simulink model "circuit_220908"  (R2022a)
settings: Solver=VariableStepAuto  StartTime=-D+0.1e-6  StopTime=34e-6  FixedStep=1e-3  MaxStep=0.1e-6  RelTol=1e-3
model workspace (MATLAB code in the model file):
  sGeo = CreateGeometry()
  sConst = CreateConstants()
libraries: fl_lib x14, nesl_utility x3, ee_lib x1

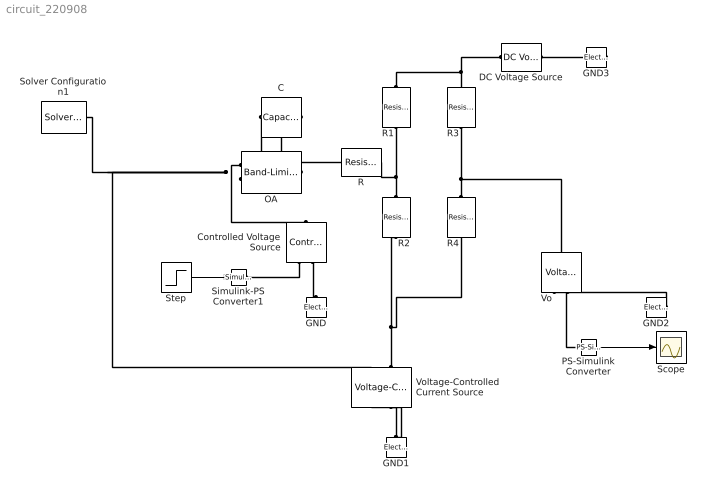
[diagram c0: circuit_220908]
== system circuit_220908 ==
  C : fl_lib/Electrical/Electrical Elements/Capacitor  c=20 nF  r=0 Ohm  g=0 1/Ohm  i_specify=off  i_priority=None  i=0 A  i_nominal_specify=off  i_nominal_unit=A  i_nominal_value=1  v_specify=off  v_priority=None  v=0 V  v_nominal_specify=off  v_nominal_unit=V  v_nominal_value=1  vc_specify=off  vc_priority=High  vc=0 V  vc_nominal_specify=off  vc_nominal_unit=V  vc_nominal_value=1
  Controlled Voltage Source : fl_lib/Electrical/Electrical Sources/Controlled Voltage Source
  DC Voltage Source : fl_lib/Electrical/Electrical Sources/DC Voltage Source  v0=10 V
  GND{,1..3} (4 alike) : fl_lib/Electrical/Electrical Elements/Electrical Reference
  OA : ee_lib/Integrated Circuits/Band-Limited Op-Amp  A=1000000  Rin=1e9 Ohm  Rout=0 Ohm  Vmin=-15 V  Vmax=15 V  Vdotmax=1000000 V/s  f=2 Hz  V0=0 V
  PS-Simulink Converter : nesl_utility/PS-Simulink Converter  PhysicalDomain=network_engine_domain  SubClassName=ps_output  LeftPortType=input  RightPortType=output  PseudoPeriodic=off  Frequencies=[]  VectorFormat=1-D array  Unit=inherit  AffineConversion=off
  R : fl_lib/Electrical/Electrical Elements/Resistor  R=100 kOhm  i_specify=off  i_priority=None  i=0 A  i_nominal_specify=off  i_nominal_unit=A  i_nominal_value=1  v_specify=off  v_priority=None  v=0 V  v_nominal_specify=off  v_nominal_unit=V  v_nominal_value=1
  R{1..4} (4 alike) : fl_lib/Electrical/Electrical Elements/Resistor  R=350 Ohm  i_specify=off  i_priority=None  i=0 A  i_nominal_specify=off  i_nominal_unit=A  i_nominal_value=1  v_specify=off  v_priority=None  v=0 V  v_nominal_specify=off  v_nominal_unit=V  v_nominal_value=1
  Scope : Scope
  Simulink-PS Converter1 : nesl_utility/Simulink-PS Converter  PhysicalDomain=network_engine_domain  SubClassName=ps_input  LeftPortType=input  RightPortType=output  PseudoPeriodic=off  Frequencies=[]  NoiseDistribution=none  NoiseParameters=[]  Unit=1  AffineConversion=off  FilteringAndDerivatives=provide  SimscapeFilterOrder=1  InputFilterTimeConstant=0.001  UdotUserProvided=0
  Solver Configuration1 : nesl_utility/Solver Configuration  PhysicalDomain=network_engine_domain  SubClassName=solver  LeftPortType=input  RightPortType=generic  Tones=[]  Harmonics=[]  SimulateNoise=off  Profile=off  UseLocalSampling=off  EnableSwitchedLinearOptims=on  FrequencyDomain=off  UseCCode=off  RelTol=0.001  AbsTol=1e-06  MinStep=1e-09  ToWorkspace=off  RevertToSquareIcSolve=off  NumHomotopyIterations=100  PhasorMode=off  PhasorModeNumHarmonics=1  IndexReductionMethod=DerivativeReplacement  DoDC=off  ResidualTolerance=1e-09  UseLocalSolver=off  LocalSolverChoice=NE_BACKWARD_EULER_ADVANCER  LocalSolverSampleTime=0.001  DoFixedCost=off  MaxNonlinIter=3  MaxModeIter=2  ComputeImpulses=off  ImpulseIterations=2  LinearAlgebra=Sparse  LinearAlgebraNumThread=0  EquationFormulation=NE_TIME_EF  DelaysMemoryBudget=1024  AutomaticFiltering=on  FilteringTimeConstant=0.001  PartitionStorageMethod=AS_NEEDED  PartitionMemoryBudget=1024  PartitionMethod=FAST
  Step : Step  SampleTime=0
  Vo : fl_lib/Electrical/Electrical Sensors/Voltage Sensor
  Voltage-Controlled Current Source : fl_lib/Electrical/Electrical Sources/Voltage-Controlled Current Source  K=1 S  v1_specify=off  v1_priority=None  v1=0 V  v1_nominal_specify=off  v1_nominal_unit=V  v1_nominal_value=1  i2_specify=off  i2_priority=None  i2=0 A  i2_nominal_specify=off  i2_nominal_unit=A  i2_nominal_value=1
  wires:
  Step/1 -> Simulink-PS Converter1/1
  PS-Simulink Converter/1 -> Scope/1
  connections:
  PS-Simulink Converter/LConn1 -- Vo/RConn1
  Controlled Voltage Source/RConn1 -- Simulink-PS Converter1/RConn1
  Controlled Voltage Source/RConn2 -- GND/LConn1
  C/RConn1 -- Solver Configuration1/RConn1 -- Voltage-Controlled Current Source/LConn1 -- OA/RConn1
  C/LConn1 -- R/LConn1 -- OA/LConn2
  OA/LConn1 -- Controlled Voltage Source/LConn1
  R2/RConn1 -- R/RConn1 -- R1/LConn1
  Voltage-Controlled Current Source/LConn2 -- R4/LConn1 -- R2/LConn1
  GND1/LConn1 -- Voltage-Controlled Current Source/RConn1 -- Voltage-Controlled Current Source/RConn2
  R4/RConn1 -- Vo/LConn1 -- R3/LConn1
  GND2/LConn1 -- Vo/RConn2
  R1/RConn1 -- R3/RConn1 -- DC Voltage Source/LConn1
  GND3/LConn1 -- DC Voltage Source/RConn1
